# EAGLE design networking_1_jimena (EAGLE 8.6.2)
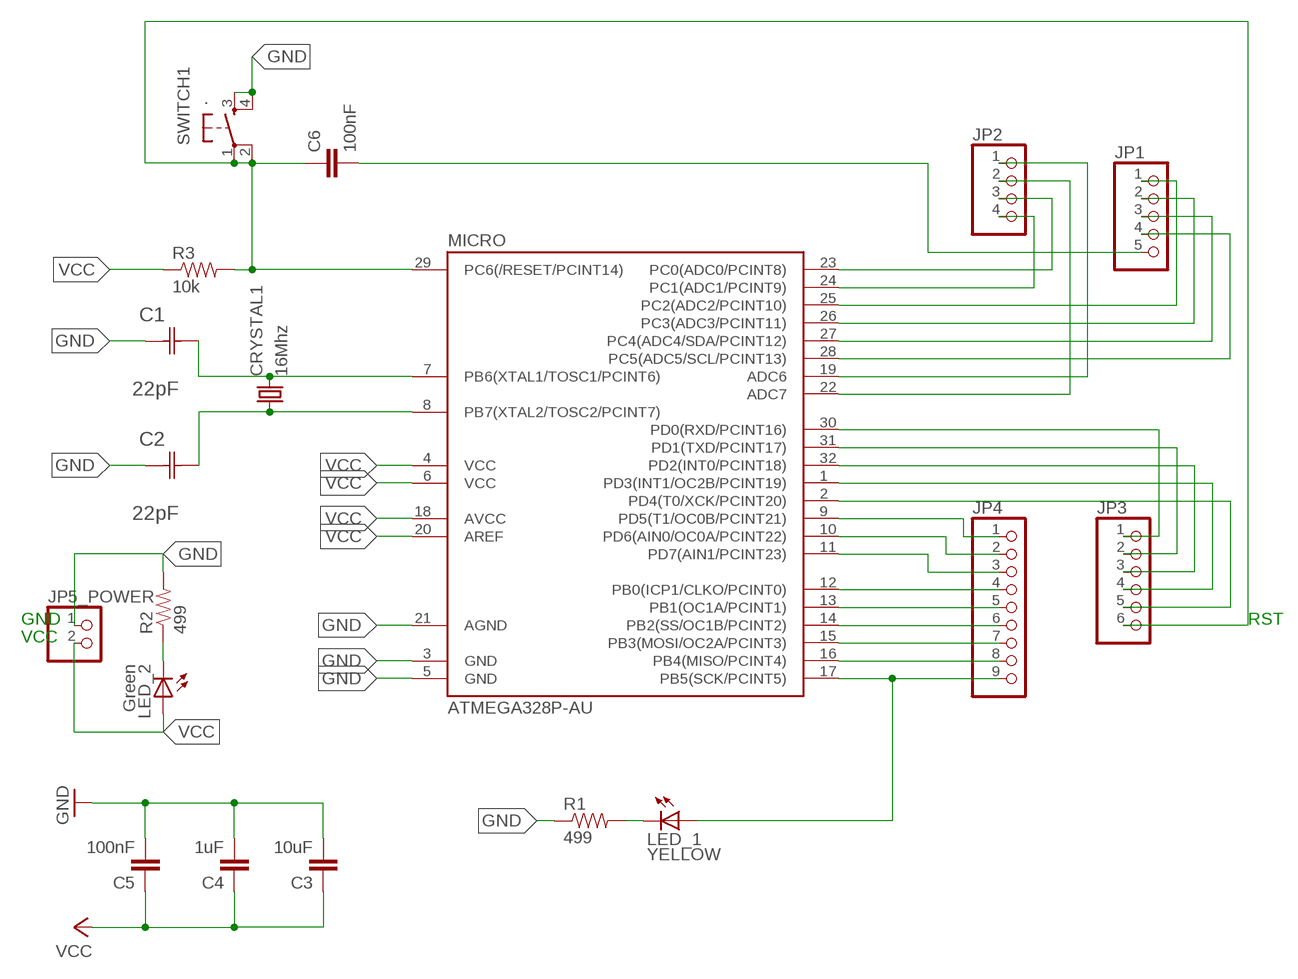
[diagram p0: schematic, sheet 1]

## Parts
C1  22pF  0612ZC225MAT2A  [CAPC3216X178N]
C2  22pF  0612ZC225MAT2A  [CAPC3216X178N]
C3  10uF  CAP1206  [1206]
C4  1uF  CAP1206  [1206]
C5  100nF  CAP1206  [1206]
C6  100nF  CAP1206  [1206]
CRYSTAL1  16Mhz  CSM-7X-DU  [CSM-7X-DU]
JP1  PINHD-1X5  [1X05]
JP2  PINHD-1X4  [1X04]
JP3  PINHD-1X6  [1X06]
JP4  PINHD-1X9  [1X09]
JP5_POWER  PINHD-1X2  [1X02]
LED_1  YELLOW  LED1206  [1206]
LED_2  Green  LED1206  [1206]
MICRO  ATMEGA328P-AU  ATMEGA48/88/168-AU  [TQFP32-08]
R1  499  RESISTOR1206  [1206]
R2  499  RESISTOR1206  [1206]
R3  10k  RESISTOR1206  [1206]
SWITCH1  .  6MM_SWITCH6MM_SWITCH  [6MM_SWITCH]

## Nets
GND: C1.1(C1) C2.1(C1) C3.2 C4.2 C5.2 JP5_POWER.1 MICRO.3(GND) MICRO.5(GND) MICRO.21(AGND) R1.1 R2.2 SWITCH1.3(S) SWITCH1.4(S1)
N$1: JP4.1 MICRO.9(PD5(T1/OC0B/PCINT21))
N$2: C1.2(C2) CRYSTAL1.2 MICRO.7(PB6(XTAL1/TOSC1/PCINT6))
N$3: C6.2 JP1.5
N$4: JP4.2 MICRO.10(PD6(AIN0/OC0A/PCINT22))
N$5: JP4.3 MICRO.11(PD7(AIN1/PCINT23))
N$6: JP4.4 MICRO.12(PB0(ICP1/CLKO/PCINT0))
N$7: JP4.5 MICRO.13(PB1(OC1A/PCINT1))
N$8: JP4.6 MICRO.14(PB2(SS/OC1B/PCINT2))
N$9: C2.2(C2) CRYSTAL1.1 MICRO.8(PB7(XTAL2/TOSC2/PCINT7))
N$10: JP4.7 MICRO.15(PB3(MOSI/OC2A/PCINT3))
N$11: JP4.8 MICRO.16(PB4(MISO/PCINT4))
N$12: JP4.9 LED_1.1(A) MICRO.17(PB5(SCK/PCINT5))
N$13: JP2.1 MICRO.19(ADC6)
N$14: JP2.2 MICRO.22(ADC7)
N$15: JP2.3 MICRO.23(PC0(ADC0/PCINT8))
N$16: JP2.4 MICRO.24(PC1(ADC1/PCINT9))
N$17: JP1.1 MICRO.25(PC2(ADC2/PCINT10))
N$18: JP1.2 MICRO.26(PC3(ADC3/PCINT11))
N$19: JP1.3 MICRO.27(PC4(ADC4/SDA/PCINT12))
N$20: JP3.1 MICRO.30(PD0(RXD/PCINT16))
N$21: JP3.2 MICRO.31(PD1(TXD/PCINT17))
N$22: JP3.3 MICRO.32(PD2(INT0/PCINT18))
N$23: JP3.4 MICRO.1(PD3(INT1/OC2B/PCINT19))
N$24: JP3.5 MICRO.2(PD4(T0/XCK/PCINT20))
N$25: JP1.4 MICRO.28(PC5(ADC5/SCL/PCINT13))
N$26: LED_2.2(C) R2.1
N$27: LED_1.2(C) R1.2
N$28: C6.1 JP3.6 MICRO.29(PC6(/RESET/PCINT14)) R3.2 SWITCH1.1(P) SWITCH1.2(P1)
VCC: C3.1 C4.1 C5.1 JP5_POWER.2 LED_2.1(A) MICRO.4(VCC) MICRO.6(VCC) MICRO.18(AVCC) MICRO.20(AREF) R3.1

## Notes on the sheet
- GND | RST
- VCC

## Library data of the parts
C1 C2 = AVX_By_element14_Batch_1:0612ZC225MAT2A: Capacitor 1206; MPN: 0612ZC225MAT2A; OC_FARNELL: -; OC_NEWARK: 12N3209; SUPPLIER: AVX; TOLERANCE: ±20%; VALUE: 2.2µF; VOLTAGERATING: 10V
C3-C6 = 01_SparkFun:CAP: Capacitor
CRYSTAL1 = 01_FAB_Hello:CSM-7X-DU: SMD CRYSTAL; OC_FARNELL: unknown; OC_NEWARK: unknown
JP1 = pinhead:PINHD-1X5: PIN HEADER
JP2 = pinhead:PINHD-1X4: PIN HEADER
JP3 = pinhead:PINHD-1X6: PIN HEADER
JP4 = pinhead:PINHD-1X9: PIN HEADER
JP5_POWER = pinhead:PINHD-1X2: PIN HEADER
LED_1 LED_2 = 01_FAB_Hello:LED
MICRO = atmega8:ATMEGA48/88/168
R1-R3 = 01_SparkFun:RESISTOR: Resistor
SWITCH1 = 01_FAB_Hello:6MM_SWITCH: OMRON SWITCH

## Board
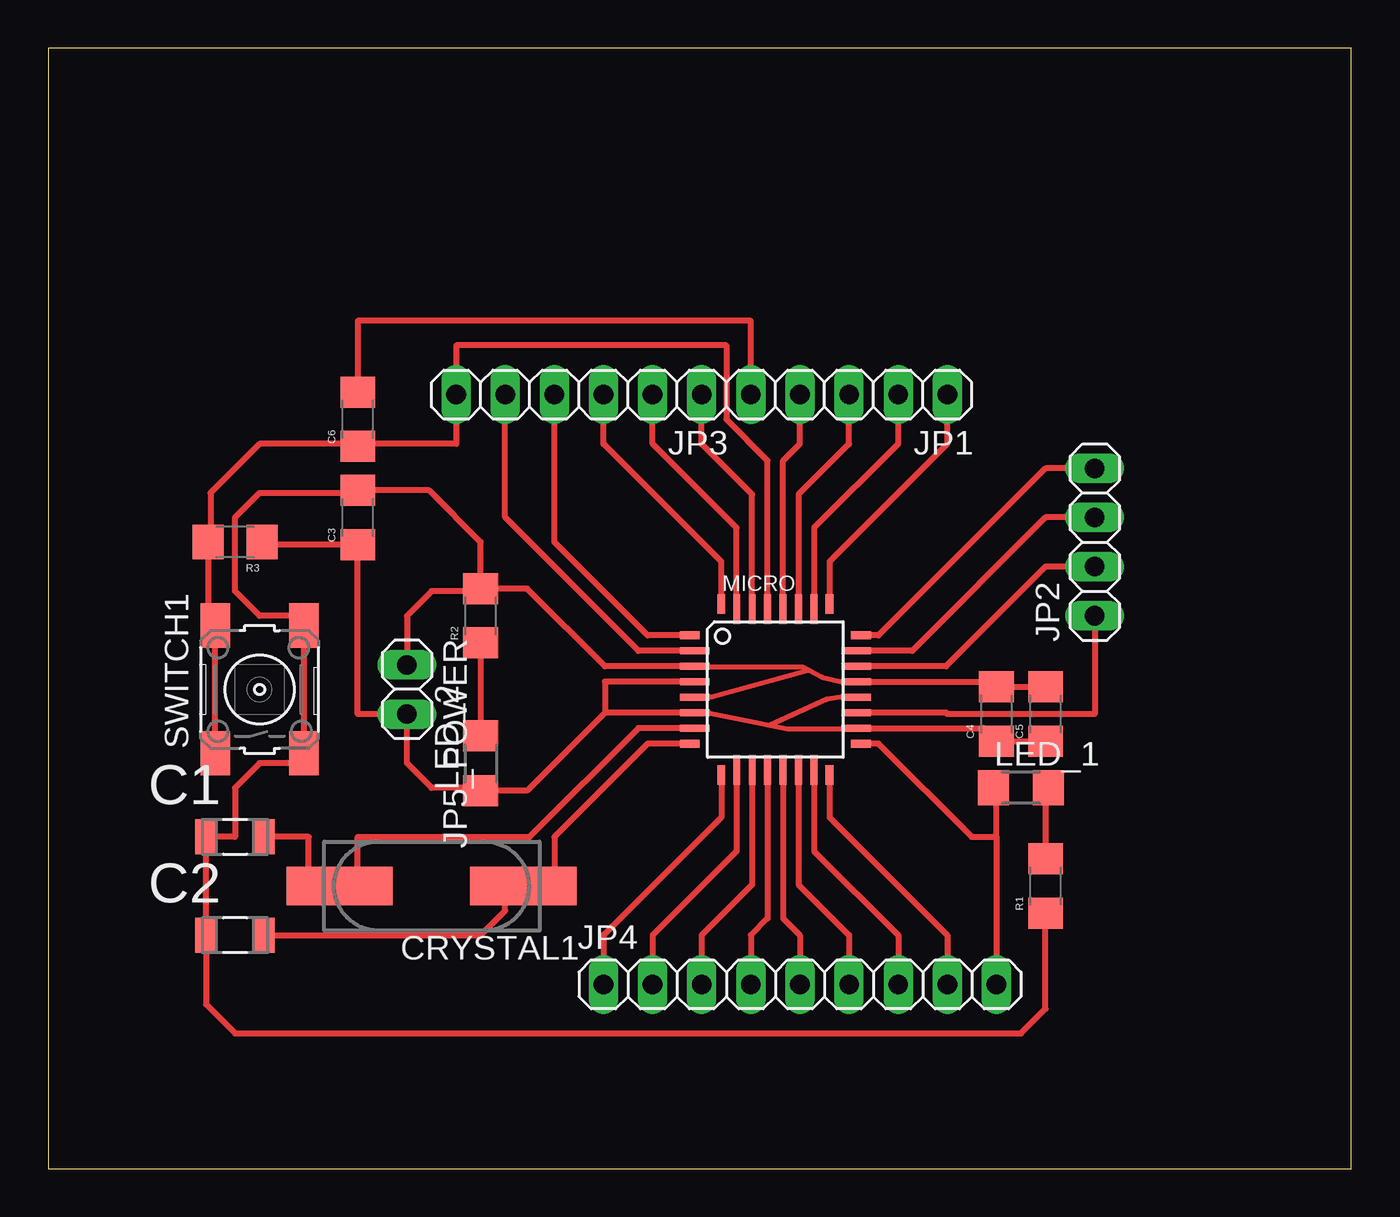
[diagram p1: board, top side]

Size 67.36 x 57.9 mm. Coordinates in mm from the lower left corner, seen from the top.
Outline: 0,0 67.36,0 67.36,57.9 0,57.9 0,0
Copper layers (1*16): Top 0.035mm / dielectric 1.5mm / Bottom 0.035mm
Design rules "default": minimum track width 10mil, minimum drill 24mil, track to track 8mil, track to pad 8mil, pad to pad 8mil, via to via 8mil, smd to smd 8mil, copper to edge 40mil, drill to drill 8mil, minimum pad ring 10mil, minimum via ring 8mil, stop-mask expansion 4mil, vias tented up to drill 0mil, thermal gap 10mil

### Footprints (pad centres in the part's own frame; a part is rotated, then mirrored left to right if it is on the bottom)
CAPC3216X178N = smd 1.118 x 1.803: 1 -1.499,0; 2 1.499,0
1206 = smd 1.6 x 1.8: 1 -1.4,0; 2 1.4,0
CSM-7X-DU = smd 5.5 x 2: 1 -4.75,0; 2 4.75,0
1X05 = drill 1.016 long: 1 -5.08,0; 2 -2.54,0; 3 0,0; 4 2.54,0; 5 5.08,0
1X04 = drill 1.016 long: 1 -3.81,0; 2 -1.27,0; 3 1.27,0; 4 3.81,0
1X06 = drill 1.016 long: 1 -6.35,0; 2 -3.81,0; 3 -1.27,0; 4 1.27,0; 5 3.81,0; 6 6.35,0
1X09 = drill 1.016 long: 1 -10.16,0; 2 -7.62,0; 3 -5.08,0; 4 -2.54,0; 5 0,0; 6 2.54,0; 7 5.08,0; 8 7.62,0; 9 10.16,0
1X02 = drill 1.016 long: 1 -1.27,0; 2 1.27,0
1206' = smd 1.6 x 1.803: 1 -1.422,0; 2 1.422,0
TQFP32-08 = smd 1.016 x 0.406: 1 -4.42,2.8; 8 -4.42,-2.8; 17 4.42,-2.8; 24 4.42,2.8 | smd 1.524 x 0.356: 2 -4.166,2; 3 -4.166,1.2; 4 -4.166,0.4; 5 -4.166,-0.4; 6 -4.166,-1.2; 7 -4.166,-2; 18 4.166,-2; 19 4.166,-1.2; 20 4.166,-0.4; 21 4.166,0.4; 22 4.166,1.2; 23 4.166,2 | smd 0.406 x 1.016: 9 -2.8,-4.42; 16 2.8,-4.42; 25 2.8,4.42; 32 -2.8,4.42 | smd 0.356 x 1.524: 10 -2,-4.166; 11 -1.2,-4.166; 12 -0.4,-4.166; 13 0.4,-4.166; 14 1.2,-4.166; 15 2,-4.166; 26 2,4.166; 27 1.2,4.166; 28 0.4,4.166; 29 -0.4,4.166; 30 -1.2,4.166; 31 -2,4.166
6MM_SWITCH = smd 2.286 x 1.524: 1 -3.302,2.286; 2 3.302,2.286; 3 -3.302,-2.286; 4 3.302,-2.286

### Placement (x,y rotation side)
C1  9.65,17.14 0 top
C2  9.65,12.07 0 top
C3  16,33.66 90 top
C4  49.02,23.5 90 top
C5  51.56,23.5 90 top
C6  16,38.73 90 top
CRYSTAL1  19.81,14.61 180 top
JP1  41.4,40.01 180 top
JP2  54.1,32.39 90 top
JP3  27.43,40.01 180 top
JP4  38.86,9.53 0 top
JP5_POWER  18.54,24.77 270 top
LED_1  YELLOW  [1206']  50.29,19.69 0 top
LED_2  Green  [1206']  22.35,20.96 90 top
MICRO  37.59,24.77 0 top
R1  51.56,14.61 90 top
R2  22.35,28.57 90 top
R3  9.65,32.39 180 top
SWITCH1  10.92,24.77 90 top

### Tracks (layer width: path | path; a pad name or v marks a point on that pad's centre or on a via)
GND
  Top 0.254: MICRO.3 33.45,25.94 38.98,25.94 | 38.98,25.94 40,25.4 41.15,25.15 | 34.04,24.38 34.29,24.38 39.17,25.73 | 39.17,25.73 39.3,25.77 | 38.98,25.94 39.17,25.73
  Top 0.305: MICRO.5 | MICRO.21 | 33.43,24.38 MICRO.5 | 34.04,24.38 MICRO.5 | MICRO.21 41.15,25.15 | MICRO.21 48.75,25.16 C4.2 C5.2 | R1.1 51.56,8.26 50.29,6.99 9.65,6.99 8.15,8.48 C2.1 C1.1 9.65,17.14 9.65,19.69 10.92,20.96 12.7,20.96 13.08,21.34 SWITCH1.3 SWITCH1.4 13.21,28.57 10.92,28.57 9.65,29.84 9.65,33.66 10.92,34.92 16,34.92 C3.2 19.68,35.05 22.35,32.39 R2.2 | MICRO.3 28.77,25.96 24.76,29.98 R2.2 | R2.2 22.22,29.84 19.81,29.84 18.54,28.57 JP5_POWER.1
N$1
  Top 0.305: MICRO.9 34.79,18.16 28.7,12.07 JP4.1
N$2
  Top 0.305: MICRO.7 30.51,22.77 24.89,17.14 16,17.14 16,15.54 CRYSTAL1.2 13.46,14.61 13.46,17.14 C1.2
N$3
  Top 0.305: JP1.5 36.32,43.81 16,43.81 C6.2
N$4
  Top 0.305: MICRO.10 35.59,16.41 31.24,12.07 JP4.2
N$5
  Top 0.305: MICRO.11 36.39,14.68 33.78,12.07 JP4.3
N$6
  Top 0.305: MICRO.12 37.19,12.94 36.32,12.07 JP4.4
N$7
  Top 0.305: MICRO.13 37.99,12.94 38.86,12.07 JP4.5
N$8
  Top 0.305: MICRO.14 38.79,14.68 41.4,12.07 JP4.6
N$9
  Top 0.305: C2.2 22.35,12.07 23.62,13.34 23.62,14.61 CRYSTAL1.1 26.16,14.61 26.16,17.14 30.98,21.96 MICRO.8
N$10
  Top 0.305: MICRO.15 39.59,16.41 43.94,12.07 JP4.7
N$11
  Top 0.305: MICRO.16 40.39,18.16 46.48,12.07 JP4.8
N$12
  Top 0.305: MICRO.17 42.93,21.96 47.75,17.14 49.02,17.14 | 49.02,17.14 49.02,19.53 LED_1.1 | 49.02,17.14 JP4.9
N$13
  Top 0.305: JP2.1 54.1,23.5 46.48,23.5 46.41,23.57 MICRO.19
N$14
  Top 0.305: MICRO.22 46.41,25.96 51.56,31.12 JP2.2
N$15
  Top 0.305: JP2.3 51.56,33.66 44.67,26.77 MICRO.23
N$16
  Top 0.305: JP2.4 51.56,36.2 42.93,27.57 MICRO.24
N$17
  Top 0.305: MICRO.25 40.39,31.38 46.48,37.47 JP1.1
N$18
  Top 0.305: MICRO.26 39.59,33.12 43.94,37.47 JP1.2
N$19
  Top 0.305: MICRO.27 38.79,34.86 41.4,37.47 JP1.3
N$20
  Top 0.305: MICRO.30 36.39,34.86 33.78,37.47 JP3.1
N$21
  Top 0.305: MICRO.31 35.59,33.12 31.24,37.47 JP3.2
N$22
  Top 0.305: MICRO.32 34.79,31.38 28.7,37.47 JP3.3
N$23
  Top 0.305: MICRO.1 30.98,27.57 26.16,32.39 JP3.4
N$24
  Top 0.305: MICRO.2 30.51,26.77 23.62,33.66 JP3.5
N$25
  Top 0.305: MICRO.28 37.99,36.59 38.86,37.47 JP1.4
N$26
  Top 0.305: R2.1 LED_2.2 22.35,22.23
N$27
  Top 0.305: LED_1.2 51.56,19.53 R1.2
N$28
  Top 0.305: 37.21,28.93 MICRO.29 37.19,36.59 35.05,38.73 35.05,42.55 21.08,42.55 JP3.6 21.08,37.47 16,37.47 15.94,37.4 | SWITCH1.1 SWITCH1.2 8.25,28.45 R3.2 8.38,32.52 8.38,34.92 10.92,37.47 15.87,37.47 15.94,37.4 | C6.1 15.94,37.4
VCC
  Top 0.254: 34.11,23.57 36.57,23.07 37.32,22.92 | 37.32,22.92 38.23,22.73 41.76,22.73 | MICRO.20 41.15,24.37 41.15,24.38 40.26,24.26 37.32,22.92
  Top 0.305: MICRO.18 | MICRO.20 41.15,24.38 | 41.76,22.73 MICRO.18 | 34.11,23.57 MICRO.6 28.77,23.57 | MICRO.18 48.35,22.77 C4.1 C5.1 | 28.77,23.57 24.74,19.53 LED_2.1 22.2,19.69 19.81,19.69 18.54,20.96 JP5_POWER.2 16,23.5 C3.1 11.18,32.25 R3.1 | MICRO.4 28.77,25.16 28.77,23.57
